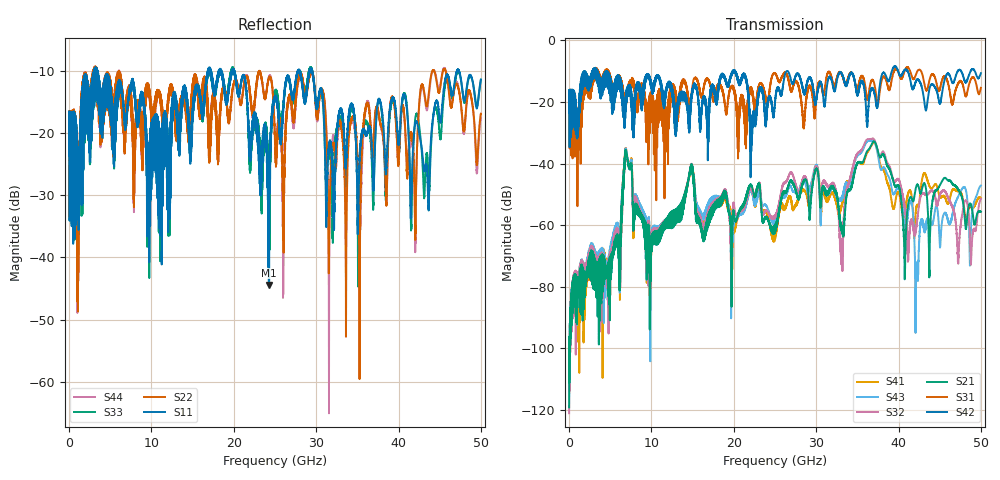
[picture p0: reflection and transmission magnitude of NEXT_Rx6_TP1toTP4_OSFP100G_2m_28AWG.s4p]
! Touchstone data
! Created: 27-Feb-2019 by IdEM 12 (12.1.0)
! COMMENTS
!  Created Wed Feb 27 12:03:36 2019
!  64 Port Network Data from SP1.SP block
!  freq  magS1_1  angS1_1  magS1_2  angS1_2  magS1_3  angS1_3  magS1_4  angS1_4
!  magS1_5  angS1_5  magS1_6  angS1_6  magS1_7  angS1_7  magS1_8  angS1_8
!  magS1_9  angS1_9  magS1_10  angS1_10  magS1_11  angS1_11  magS1_12  angS1_12
!  magS1_13  angS1_13  magS1_14  angS1_14  magS1_15  angS1_15  magS1_16  angS1_16
!  magS1_17  angS1_17  magS1_18  angS1_18  magS1_19  angS1_19  magS1_20  angS1_20
!  magS1_21  angS1_21  magS1_22  angS1_22  magS1_23  angS1_23  magS1_24  angS1_24
!  magS1_25  angS1_25  magS1_26  angS1_26  magS1_27  angS1_27  magS1_28  angS1_28
!  magS1_29  angS1_29  magS1_30  angS1_30  magS1_31  angS1_31  magS1_32  angS1_32
!  magS1_33  angS1_33  magS1_34  angS1_34  magS1_35  angS1_35  magS1_36  angS1_36
!  magS1_37  angS1_37  magS1_38  angS1_38  magS1_39  angS1_39  magS1_40  angS1_40
!  magS1_41  angS1_41  magS1_42  angS1_42  magS1_43  angS1_43  magS1_44  angS1_44
!  magS1_45  angS1_45  magS1_46  angS1_46  magS1_47  angS1_47  magS1_48  angS1_48
!  magS1_49  angS1_49  magS1_50  angS1_50  magS1_51  angS1_51  magS1_52  angS1_52
!  magS1_53  angS1_53  magS1_54  angS1_54  magS1_55  angS1_55  magS1_56  angS1_56
!  magS1_57  angS1_57  magS1_58  angS1_58  magS1_59  angS1_59  magS1_60  angS1_60
!  magS1_61  angS1_61  magS1_62  angS1_62  magS1_63  angS1_63  magS1_64  angS1_64
!  magS2_1  angS2_1  magS2_2  angS2_2  magS2_3  angS2_3  magS2_4  angS2_4
!  magS2_5  angS2_5  magS2_6  angS2_6  magS2_7  angS2_7  magS2_8  angS2_8
!  magS2_9  angS2_9  magS2_10  angS2_10  magS2_11  angS2_11  magS2_12  angS2_12
!  magS2_13  angS2_13  magS2_14  angS2_14  magS2_15  angS2_15  magS2_16  angS2_16
!  magS2_17  angS2_17  magS2_18  angS2_18  magS2_19  angS2_19  magS2_20  angS2_20
!  magS2_21  angS2_21  magS2_22  angS2_22  magS2_23  angS2_23  magS2_24  angS2_24
!  magS2_25  angS2_25  magS2_26  angS2_26  magS2_27  angS2_27  magS2_28  angS2_28
!  magS2_29  angS2_29  magS2_30  angS2_30  magS2_31  angS2_31  magS2_32  angS2_32
!  magS2_33  angS2_33  magS2_34  angS2_34  magS2_35  angS2_35  magS2_36  angS2_36
!  magS2_37  angS2_37  magS2_38  angS2_38  magS2_39  angS2_39  magS2_40  angS2_40
!  magS2_41  angS2_41  magS2_42  angS2_42  magS2_43  angS2_43  magS2_44  angS2_44
!  magS2_45  angS2_45  magS2_46  angS2_46  magS2_47  angS2_47  magS2_48  angS2_48
!  magS2_49  angS2_49  magS2_50  angS2_50  magS2_51  angS2_51  magS2_52  angS2_52
!  magS2_53  angS2_53  magS2_54  angS2_54  magS2_55  angS2_55  magS2_56  angS2_56
!  magS2_57  angS2_57  magS2_58  angS2_58  magS2_59  angS2_59  magS2_60  angS2_60
!  magS2_61  angS2_61  magS2_62  angS2_62  magS2_63  angS2_63  magS2_64  angS2_64
!  magS3_1  angS3_1  magS3_2  angS3_2  magS3_3  angS3_3  magS3_4  angS3_4
!  magS3_5  angS3_5  magS3_6  angS3_6  magS3_7  angS3_7  magS3_8  angS3_8
!  magS3_9  angS3_9  magS3_10  angS3_10  magS3_11  angS3_11  magS3_12  angS3_12
!  magS3_13  angS3_13  magS3_14  angS3_14  magS3_15  angS3_15  magS3_16  angS3_16
!  magS3_17  angS3_17  magS3_18  angS3_18  magS3_19  angS3_19  magS3_20  angS3_20
!  magS3_21  angS3_21  magS3_22  angS3_22  magS3_23  angS3_23  magS3_24  angS3_24
!  magS3_25  angS3_25  magS3_26  angS3_26  magS3_27  angS3_27  magS3_28  angS3_28
!  magS3_29  angS3_29  magS3_30  angS3_30  magS3_31  angS3_31  magS3_32  angS3_32
!  magS3_33  angS3_33  magS3_34  angS3_34  magS3_35  angS3_35  magS3_36  angS3_36
!  magS3_37  angS3_37  magS3_38  angS3_38  magS3_39  angS3_39  magS3_40  angS3_40
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# Hz S MA R 50
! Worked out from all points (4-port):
!   5000 points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, 10 MHz to 50 GHz, reference 50 ohm
!   strongest paths, dB at 10 MHz, 12.51 GHz, 25.01 GHz, 37.51 GHz, 50 GHz:
!     S42: -18.1, -16.3, -19.6, -20.0, -10.7
!     S31: -18.0, -15.9, -10.7, -20.7, -15.4
!     S21: -119.2, -59.5, -62.2, -36.1, -55.6
!     S32: -121.2, -59.6, -57.6, -36.4, -51.5
!     S43: -115.7, -59.1, -58.9, -37.4, -47.1
!     S41: -114.4, -59.2, -63.2, -36.6, -51.2
!   lowest |S11| = -44.4 dB at 24.26 GHz (marker M1), VSWR 1.01, Z = 49.6 - j0.401 ohm
!   |S11| at or under -10 dB: 3.451 GHz to 16.86 GHz (13.4 GHz wide, 132 % of centre); 20.09 GHz to 27.79 GHz (7.695 GHz wide, 32.1 % of centre); 29.5 GHz to 47.1 GHz (17.61 GHz wide, 46 % of centre)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
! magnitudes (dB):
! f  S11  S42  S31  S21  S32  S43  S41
! 10 MHz  -17.7  -18.1  -18.0  -119.2  -121.2  -115.7  -114.4
! 6.04 GHz  -13.0  -13.4  -12.4  -66.0  -63.8  -62.0  -63.8
! 6.96 GHz  -17.1  -16.4  -19.0  -36.4  -36.5  -35.8  -35.6
! 9.84 GHz  -21.6  -12.4  -17.6  -72.6  -70.5  -69.0  -71.0
! 24.26 GHz  -44.4  -18.9  -18.3  -59.3  -56.3  -55.9  -58.8
! 42.22 GHz  -18.2  -12.9  -10.4  -47.0  -59.8  -73.5  -53.5
! 50 GHz  -11.4  -10.7  -15.4  -55.6  -51.5  -47.1  -51.2
